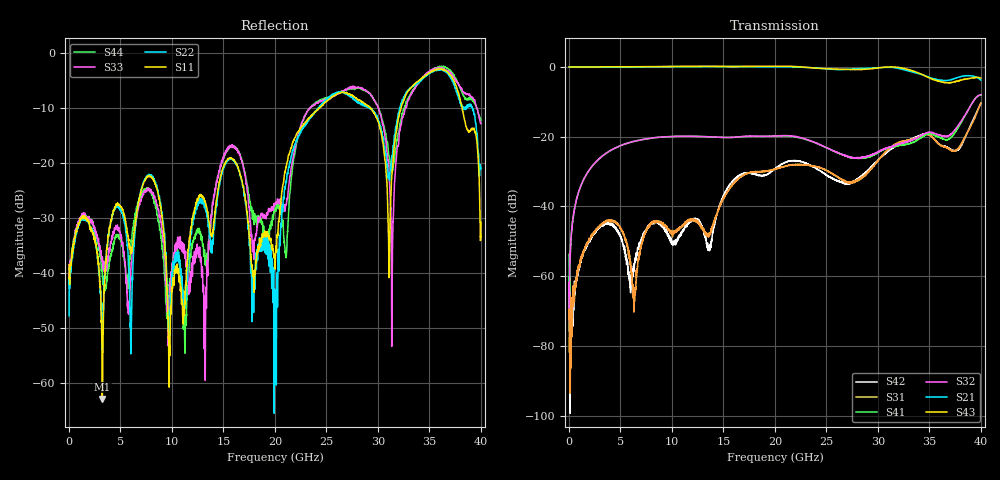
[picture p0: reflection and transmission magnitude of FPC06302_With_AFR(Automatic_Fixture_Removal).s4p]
!The following data was pulled from an Agilent PNA
!This sNp file was generated from the data in the RF Test software
!NOTE:  Smoothing/Math/Corrections applied on any given trace ARE included in the data saved here
# MHz S dB R 50
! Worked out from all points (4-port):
!   4000 points, 10 MHz to 40 GHz, reference 50 ohm
!   strongest paths, dB at 10 MHz, 10.01 GHz, 20.01 GHz, 30.01 GHz, 40 GHz:
!     S43: 0.0, 0.1, 0.1, -0.3, -3.3
!     S21: -0.1, 0.0, 0.0, -0.3, -3.9
!     S32: -69.1, -20.0, -19.8, -24.4, -8.0
!     S41: -53.7, -20.0, -19.9, -24.6, -8.1
!     S31: -62.0, -47.9, -29.3, -26.9, -10.3
!     S42: -64.6, -50.1, -29.3, -26.8, -10.5
!   lowest |S11| = -62.8 dB at 3.23 GHz (marker M1), VSWR 1.00, Z = 50 + j0.0716 ohm
!   |S11| at or under -10 dB: start of sweep to 24.33 GHz; 29.28 GHz to 32.25 GHz (2.97 GHz wide, 9.65 % of centre); 38.17 GHz to end of sweep
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10  -38.46 -175.9  -0.07 0.0  -60.64 -146.9  -64.73 -149.2
    -0.08 -0.1  -47.74 -158.8  -59.45 79.9  -59.27 74.5
    -61.99 176.3  -69.13 55.8  -38.40 -133.2  -0.09 0.1
    -53.75 69.7  -64.60 -55.4  -0.05 0.4  -39.17 -146.8
3230  -62.81 97.9  -0.08 -42.2  -44.86 50.3  -25.65 48.3
      -0.08 -42.2  -52.90 -29.3  -25.63 47.3  -45.57 45.4
      -44.90 50.9  -25.64 47.3  -37.01 5.7  -0.03 -42.3
      -25.65 48.1  -45.49 45.9  -0.03 -42.3  -39.94 73.2
12950  -26.06 -68.4  0.05 -177.8  -46.44 78.2  -20.02 -86.4
       0.06 -177.8  -26.63 -102.5  -20.00 -89.3  -45.64 65.7
       -46.01 81.0  -20.00 -89.3  -39.32 -109.3  0.16 -178.6
       -20.02 -86.4  -46.19 65.9  0.15 -178.6  -34.70 -28.3
20080  -35.10 36.3  0.02 75.4  -29.33 -16.6  -19.88 166.5
       0.03 75.4  -44.78 -117.1  -19.84 163.3  -29.15 -6.9
       -29.29 -16.8  -19.83 163.4  -27.17 -24.6  0.14 73.1
       -19.87 166.6  -29.08 -6.6  0.13 73.2  -28.76 -8.5
23550  -11.29 112.3  -0.29 18.3  -28.40 -105.6  -21.40 104.5
       -0.29 18.3  -11.49 99.4  -21.32 99.1  -28.44 -113.2
       -28.34 -105.8  -21.33 99.6  -9.74 106.4  -0.29 15.5
       -21.37 104.7  -28.43 -113.0  -0.29 15.6  -9.77 100.5
33110  -6.46 106.6  -1.34 -156.0  -20.96 -104.9  -22.00 -104.4
       -1.35 -156.0  -6.39 111.6  -21.33 -113.0  -20.92 -101.6
       -20.96 -104.7  -21.25 -113.4  -7.85 99.0  -0.94 -161.3
       -21.95 -104.2  -20.86 -101.9  -0.94 -161.3  -7.58 105.2
40000  -30.71 -6.6  -3.83 47.1  -10.33 98.8  -8.15 -45.7
       -3.85 47.0  -20.93 3.0  -8.00 -52.5  -10.57 95.8
       -10.34 98.8  -7.99 -52.4  -12.78 -49.7  -3.25 48.9
       -8.14 -45.7  -10.54 95.7  -3.25 48.9  -12.02 -30.1
